ORGANIZATION_BLOCK OB 1
BEGIN

	// Test SFC -1: __NOP
	CALL		SFC -1


	// Test SFC 64: TIME_TCK
	CALL		SFC 64 (
		RET_VAL		:= MD 0
	)
	__SLEEP		100
	CALL		SFC 64 (
		RET_VAL		:= MD 4
	)
	L		MD 4
	L		MD 0
	-D
	UD		DW#16#7FFFFFFF
	__ASSERT>	__ACCU 1,	50
	__ASSERT<	__ACCU 1,	500

END_ORGANIZATION_BLOCK
